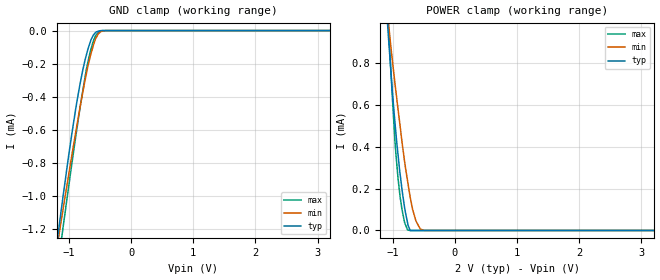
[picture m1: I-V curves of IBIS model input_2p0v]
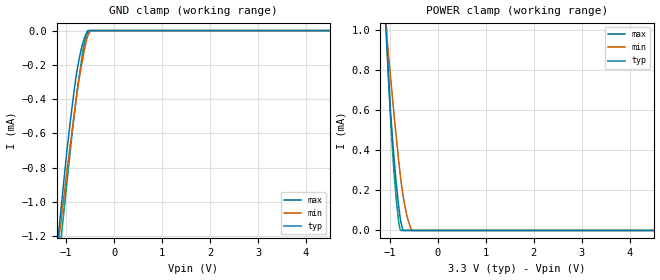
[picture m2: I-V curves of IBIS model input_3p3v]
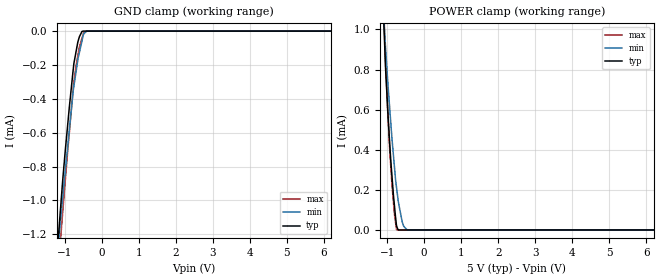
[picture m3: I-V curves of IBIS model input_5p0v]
|Texas Instruments Incorporated
|12bit, Single Channel, 80uA, 1.8V-5.5V DAC in SC70 Package
| Marketing part#   Digital Voltage Range   Package-type   #pins
| DAC7311IDCKR   1.8 to 5.5V   SC70   6
| DAC7311IDCKRG4   1.8 to 5.5V   SC70   6
| DAC7311IDCKT   1.8 to 5.5V   SC70   6
| DAC7311IDCKTG4   1.8 to 5.5V   SC70   6
[IBIS Ver]   3.2
[File name]   dac7311.ibs
|SIMDE Ver   V2.0 - 201002 - RHL4 - Build 372
[File Rev]   1.2
[Date]   07/13/2010
[Source]
|   Texas Instruments Incorporated.
|   Analog-eLab Design Center, HPA
|   12500 TI Blvd
|   Dallas, TX -75243
|   e-mail: elab_ibis@list.ti.com
|   Model generated from simulations in TISPICE
[Notes]   Revision History:
|   Rev 1.0: 06/28/2010
|   - Initial version of the model
|   - Model generated from simulations in TISPICE
|   - Model matched to SPICE simulation
|   - Model names with a trailing 3p3v contains the model for
|   3.3V [3.0V and 3.6V]. Model names with trailing 5p0v contains
|   the model for 5.0V [4.5V and 5.5V] operation.
|   - C_comp although listed in numerical order of value are obtained
|   from varying PVT conditions. For PVT conditions for each specific
|   value refer the buffer description under respective [Model]. IBIS
|   model user is responsible for using appropriate C_comp to simulate
|   for Signal Integrity.
|   Rev 1.1: 07/10/2010
|   - Added input_2p0v model to the IBIS file.
|   - Model names with a trailing 2p0v contains the model for
|   2.0V [1.8V and 2.2V].Model names with a trailing 3p3v contains
|   the model for 3.3V [3.0V and 3.6V]. Model names with trailing 5p0v
|   contains the model for 5.0V [4.5V and 5.5V] operation.
|   - Updated the package details with correct values.
|   Rev 1.2: 07/13/2010
|   - Removed data points beyond -VCCtyp and 2*VCCtyp range for IV data.
|   - Added comment that temperatures used are junction temperatures
|   - Fixed Vinl and Vinh values as per datasheet
[Disclaimer]
| This model is designed as an aid for customers of Texas Instruments.
| TI and its licensors and suppliers make no warranties, either expressed
| or implied, with respect to this  model, including the warranties of
| merchantability or fitness for a particular purpose. The model is
| provided solely on an "as is" basis. The entire risk as to its quality
| and performance is with the customer.
[Copyright]
|(C) Copyright 2010 Texas Instruments Incorporated.All rights reserved.
|   DAC7311
[Component]   DAC7311
[Manufacturer]  TI
[Package]   | 6 SC70 - DCK package
|   typ   min   max
R_pkg   0.02865   0.00688   0.05042
L_pkg   1.430605nH   1.31953nH   1.54168nH
C_pkg   0.28112pF   0.22169pF   0.34055pF
|-------------------------PINS------------------------------------------------
[Pin]  signal_name model_name   R_pin   L_pin   C_pin
1   _SYNC   INPUT   0.05036   1.43819nH   0.27388pF
2   SCLK   INPUT   0.00688   1.54168nH   0.34055pF
3   Din   INPUT   0.05002   1.31953nH   0.22169pF
4   AVDD/VREF   POWER   0.05111   1.45036nH   0.27435pF
5   GND   GND   0.00690   1.54395nH   0.34010pF
6   Vout   NC   0.05042   1.32551nH   0.22210pF
|   Model Selectors
[Model Selector]   INPUT
input_2p0v   2.0V digital input
input_3p3v   3.3V digital input
input_5p0v   5.0V digital input
| Models and submodels in the file (3): input_2p0v (Input), input_3p3v (Input), input_5p0v (Input)
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|   INPUT 2.0V Model
[Model]   input_2p0v
Model_type   Input
Vinl = 0.25
Vinh = 1.65
|   typ   min   max
|   (Nom PVT)   (Fast PVT)  (Slow PVT)
C_comp   4.846e-13   4.442e-13   5.322e-13
|Where nom PVT is Nom process, 2.0V, 25C
|Fast PVT is Strong Process, 2.2V, -40C
|Slow PVT is Weak Process,   1.8V, 125C
[Model Spec]
Vinl   0.25   0.0   0.5
Vinh   1.65   1.1   2.2
[Voltage Range]   2   1.8   2.2
|Junction temperatures are used for [Temperature Range]
[Temperature Range]   25   125   -40
[Power Clamp Reference]   2   1.8   2.2
[GND Clamp Reference]   0   0   0
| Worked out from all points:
|   GND clamp passes 1 mA (typ) near -1.09 V on its own axis
|   POWER clamp passes 1 mA (typ) near -1.09 V on its own axis
[GND Clamp]
|   Voltage   I(typ)   I(min)   I(max)
-2V       -3.727mA   -3.284mA   -4.306mA
-1.194V   -1.284mA   -1.314mA   -1.472mA
-1.131V   -1.105mA   -1.167mA   -1.291mA
-1.108V   -1.039mA   -1.113mA   -1.228mA
-944mV    -601.3uA   -732.9uA   -780.8uA
-782mV    -247.4uA   -382.5uA   -374.3uA
-684.4mV  -100.2uA   -198.4uA   -171uA
-620.6mV  -36.88uA   -107.1uA   -78.82uA
-558mV    -7.517uA   -40.41uA   -24.33uA
-486.2mV  0A         -5.532uA   -2.528uA
-416mV    0A         0A         0A
4V        0A         0A         0A
[POWER Clamp]
|   Voltage   I(typ)   I(min)   I(max)
-2V       6.043mA    4.898mA    7.255mA
-1.076V   957.6uA    1.013mA    1.02mA
-1.066V   914uA      984.4uA    963.8uA
-1.041V   809.3uA    911.5uA    822.9uA
-963.8mV  515.5uA    703uA      426.9uA
-913.2mV  358.9uA    577.7uA    246.9uA
-853.8mV  203.7uA    432.2uA    105.7uA
-761.4mV  37.48uA    237.8uA    2.937uA
-718.4mV  0A         158.5uA    0A
-628.4mV  0A         47.57uA    0A
-497mV    0A         0A         0A
4V        0A         0A         0A
|   INPUT 3.3V Model
[Model]   input_3p3v
Model_type   Input
Vinl = 0.25
Vinh = 2.35
|   typ   min   max
|   (Nom PVT)   (Fast PVT)  (Slow PVT)
C_comp   4.649e-13   4.574e-13   5.358e-13
|Where nom PVT is Nom process, 3.3V, 25C
|Fast PVT is Strong Process, 3.6V, -40C
|Slow PVT is Weak Process,   3.0V, 125C
[Model Spec]
Vinl   0.25   0.0   0.5
Vinh   2.35   1.1   3.6
[Voltage Range]   3.3   3   3.6
|Junction temperatures are used for [Temperature Range]
[Temperature Range]   25   125   -40
[Power Clamp Reference]   3.3   3   3.6
[GND Clamp Reference]   0   0   0
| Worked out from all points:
|   GND clamp passes 1 mA (typ) near -1.09 V on its own axis
|   POWER clamp passes 1 mA (typ) near -1.08 V on its own axis
[GND Clamp]
|   Voltage   I(typ)   I(min)   I(max)
-3.3V     -7.771mA   -6.523mA   -9.241mA
-1.161V   -1.192mA   -1.237mA   -1.375mA
-1.079V   -964uA     -1.045mA   -1.143mA
-983.4mV  -700.3uA   -823uA     -888.3uA
-834mV    -353.1uA   -492.4uA   -497.2uA
-785.4mV  -253uA     -389.7uA   -389.1uA
-729.3mV  -165.2uA   -285.1uA   -269.8uA
-639.6mV  -62.63uA   -141.6uA   -99.97uA
-573mV    -13.74uA   -51.62uA   -31.94uA
-549.6mV  -492.7nA   -32.71uA   -15.28uA
-486mV    0A         0A         0A
6.6V      0A         0A         0A
[POWER Clamp]
|   Voltage   I(typ)   I(min)   I(max)
-3.3V     13.63mA    10.97mA    16.39mA
-1.104V   1.1mA      1.093mA    1.198mA
-1.076V   970.6uA    1.01mA     1.029mA
-1.018V   725.9uA    845.4uA    698.9uA
-920.4mV  381.8uA    594.6uA    311.9uA
-866.4mV  234.7uA    464.3uA    151.6uA
-816mV    121uA      346.7uA    42.15uA
-778.8mV  53.33uA    267.9uA    0A
-719.4mV  0A         166.5uA    0A
-657mV    0A         85.88uA    0A
-535.2mV  0A         0A         0A
6.6V      0A         0A         0A
|   INPUT 5.0V Model
[Model]   input_5p0v
Model_type   Input
Vinl = 0.4
Vinh = 3.65
|   typ   min   max
|   (Nom PVT)   (Fast PVT)  (Slow PVT)
C_comp   4.340e-13   3.990e-13   5.354e-13
|Where nom PVT is Nom process,5.0V, 25C
|Fast PVT is Strong Process,5.5V, -40C
|Slow PVT is Weak Process,  4.5V, 125C
[Model Spec]
Vinl   0.4   0.0   0.8
Vinh   3.65   1.8   5.5
[Voltage Range]   5   4.5   5.5
|Junction temperatures are used for [Temperature Range]
[Temperature Range]   25   125   -40
[Power Clamp Reference]   5   4.5   5.5
[GND Clamp Reference]   0   0   0
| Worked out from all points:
|   GND clamp passes 1 mA (typ) near -1.09 V on its own axis
|   POWER clamp passes 1 mA (typ) near -1.08 V on its own axis
[GND Clamp]
|   Voltage   I(typ)   I(min)   I(max)
-5V       -13.07mA   -10.77mA   -15.71mA
-1.155V   -1.177mA   -1.225mA   -1.362mA
-1.079V   -959.1uA   -1.043mA   -1.144mA
-990mV    -726.1uA   -844.8uA   -903.6uA
-870mV    -444.5uA   -578.7uA   -594.1uA
-750mV    -191.7uA   -326.1uA   -301.6uA
-640mV    -62.84uA   -166.7uA   -140.6uA
-600mV    -33uA      -125.5uA   -92.78uA
-530mV    -2.078uA   -57.4uA    -41.23uA
-486.5mV  0A         -17.47uA   -11.95uA
-405.5mV  0A         0A         0A
10V       0A         0A         0A
[POWER Clamp]
|   Voltage   I(typ)   I(min)   I(max)
-5V       23.6mA     18.99mA    28.37mA
-1.205V   1.603mA    1.456mA    1.84mA
-1.071V   949.8uA    999uA      999.2uA
-1.045V   820.1uA    918.8uA    851.6uA
-990.5mV  625.8uA    762.8uA    620uA
-924.5mV  414.4uA    594uA      384.8uA
-869.5mV  270.3uA    457.4uA    226.7uA
-809mV    134.7uA    330uA      92.48uA
-745mV    20.34uA    211uA      1.195uA
-594.5mV  0A         42.39uA    0A
-451.5mV  0A         0A         0A
10V       0A         0A         0A
